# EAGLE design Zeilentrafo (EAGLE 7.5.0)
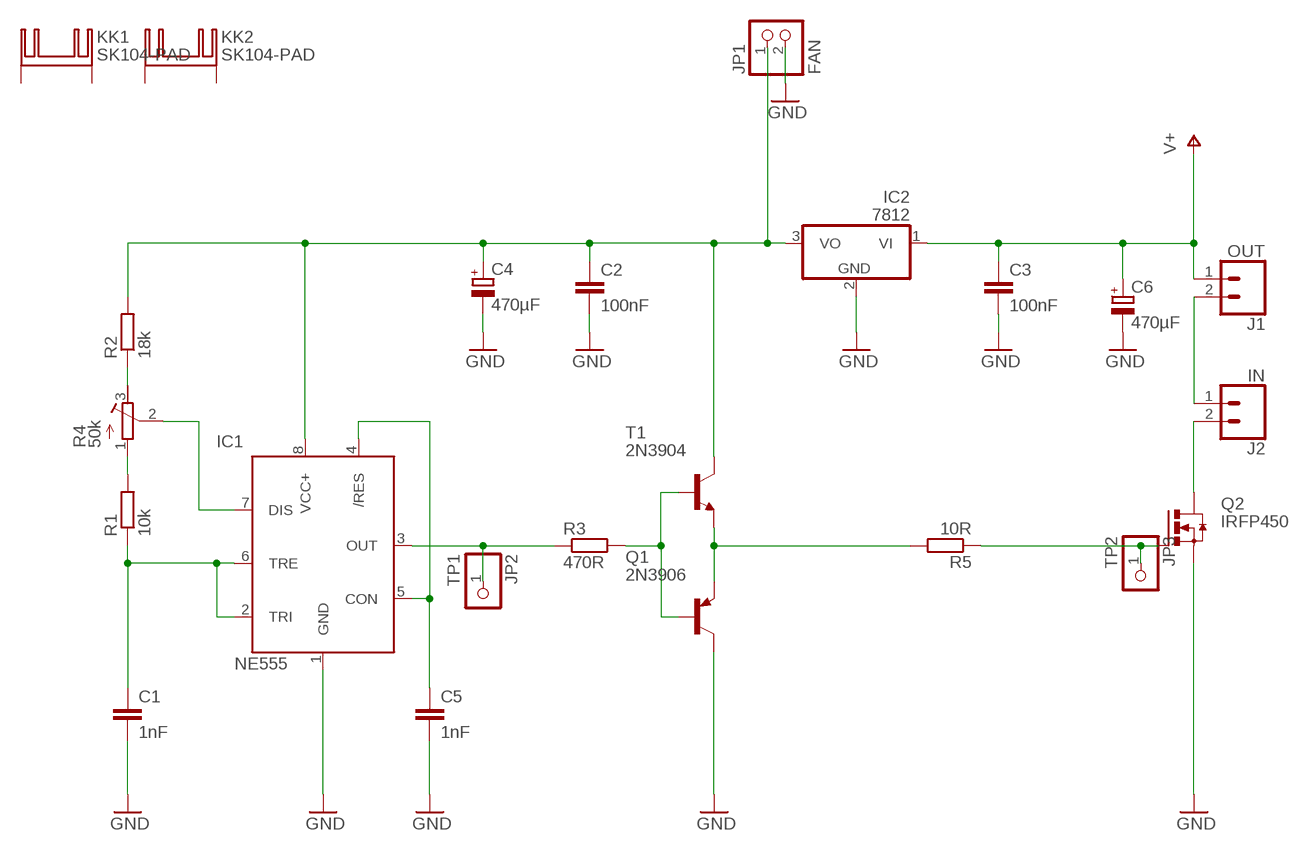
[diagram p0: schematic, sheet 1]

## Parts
C1  1nF  C-EU050-024X044  [C050-024X044]
C2  100nF  C-EU050-024X044  [C050-024X044]
C3  100nF  C-EU050-024X044  [C050-024X044]
C4  470µF  CPOL-EUE5-10.5  [E5-10,5]
C5  1nF  C-EU050-024X044  [C050-024X044]
C6  470µF  CPOL-EUE5-10.5  [E5-10,5]
IC1  NE555  [DIL-08]
IC2  7812  7812TV  [TO220V]
J1  OUT  CONN_025MM  [SCREWTERMINAL-5MM-2]
J2  IN  CONN_025MM  [SCREWTERMINAL-5MM-2]
JP1  FAN  PINHD-1X2  [1X02]
JP2  TP1  PINHD-1X1  [1X01]
JP3  TP2  PINHD-1X1  [1X01]
KK1  SK104-PAD  [SK104-PAD]
KK2  SK104-PAD  [SK104-PAD]
Q1  2N3906  [TO92]
Q2  IRFP450  IRFP240  [TO247BV]
R1  10k  R-EU_0207/12  [0207/12]
R2  18k  R-EU_0207/12  [0207/12]
R3  470R  R-EU_0207/12  [0207/12]
R4  50k  R-TRIMM3296Y  [RTRIM3296Y]
R5  10R  R-EU_0207/12  [0207/12]
T1  2N3904  [TO92]

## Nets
GND: C1.2 C2.2 C3.2 C4.- C5.2 C6.- IC1.1(GND) IC2.2(GND) JP1.2 Q1.1(C) Q2.S
N$1: C1.1 IC1.2(TRI) IC1.6(TRE) R1.1
N$2: IC1.7(DIS) R4.2(S)
N$3: R1.2 R4.1(A)
N$4: R2.1 R4.3(E)
N$5: C2.1 C4.+ IC1.8(VCC+) IC2.3(VO) JP1.1 R2.2 T1.1(C)
N$6: JP3.1 Q2.G R5.1
N$7: IC1.3(OUT) JP2.1 R3.1
N$8: Q1.2(B) R3.2 T1.2(B)
N$9: Q1.3(E) R5.2 T1.3(E)
N$10: J1.2 J2.1
N$11: C5.1 IC1.4(/RES) IC1.5(CON)
N$13: J2.2 Q2.D
V+: C3.1 C6.+ IC2.1(VI) J1.1
Unconnected: KK1.K1(K) KK1.K2(K) KK2.K1(K) KK2.K2(K)

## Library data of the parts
C1-C3 C5 = rcl_custom:C-EU: CAPACITOR, European symbol
C4 C6 = rcl_custom:CPOL-EU: POLARIZED CAPACITOR, European symbol
IC1 = st-microelectronics_custom:NE555: General purpose bipolar Timer; MF: Arrow Electronics; MPN: NE555N; OC_FARNELL: 1467742; OC_NEWARK: 89K1486
IC2 = linear:78*: Positive VOLTAGE REGULATOR Source: http://cache.national.com/ds/LM/LM78L05.pdf http://www.fairchildsemi.com/ds/LM/LM7805.pdf
J1 J2 = SparkFun-Connectors:CONN_02: Multi connection point. Often used as Generic Header-pin footprint for 0.1 inch spaced/style header connections; SF_SKU: PRT-08432
JP1 = pinhead:PINHD-1X2: PIN HEADER
JP2 JP3 = pinhead:PINHD-1X1: PIN HEADER
KK1 KK2 = heatsink_custom:SK104-PAD: HEATSINK
Q1 = transistor-pnp:2N3906: PNP Transistor
Q2 = transistor-power:IRFP240: HEXFET Power MosFet Source: http://www.irf.com/
R1-R3 R5 = rcl_custom:R-EU_: RESISTOR, European symbol
R4 = rcl:R-TRIMM: Trimm resistor
T1 = transistor:2N3904: NPN TRANSISTOR

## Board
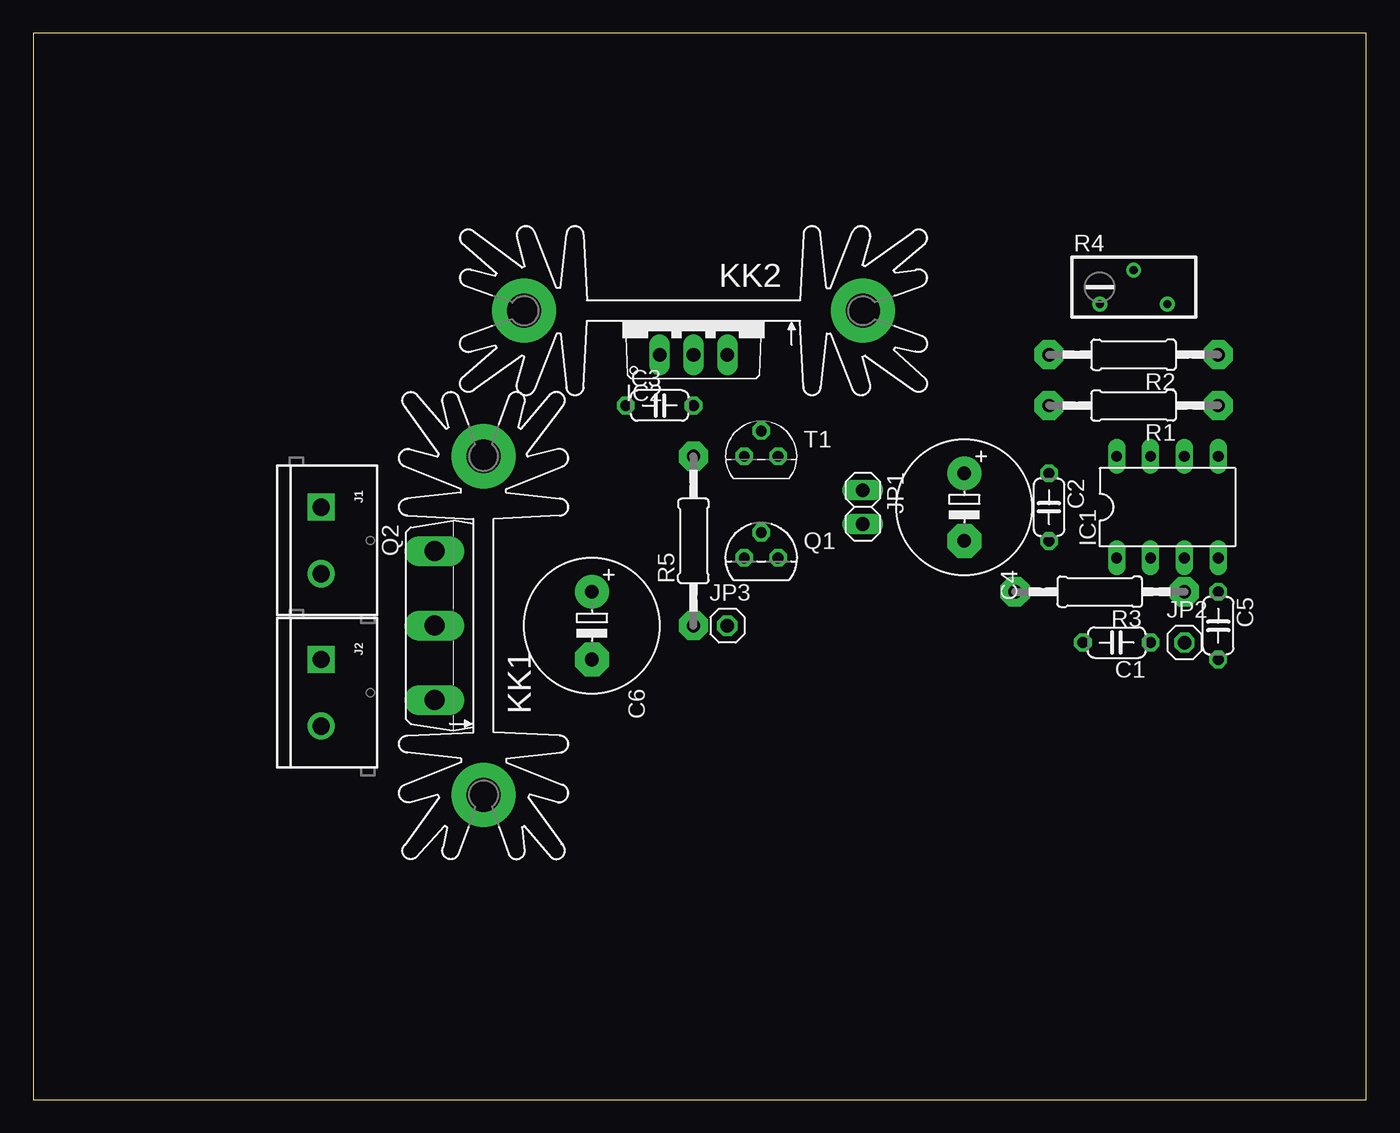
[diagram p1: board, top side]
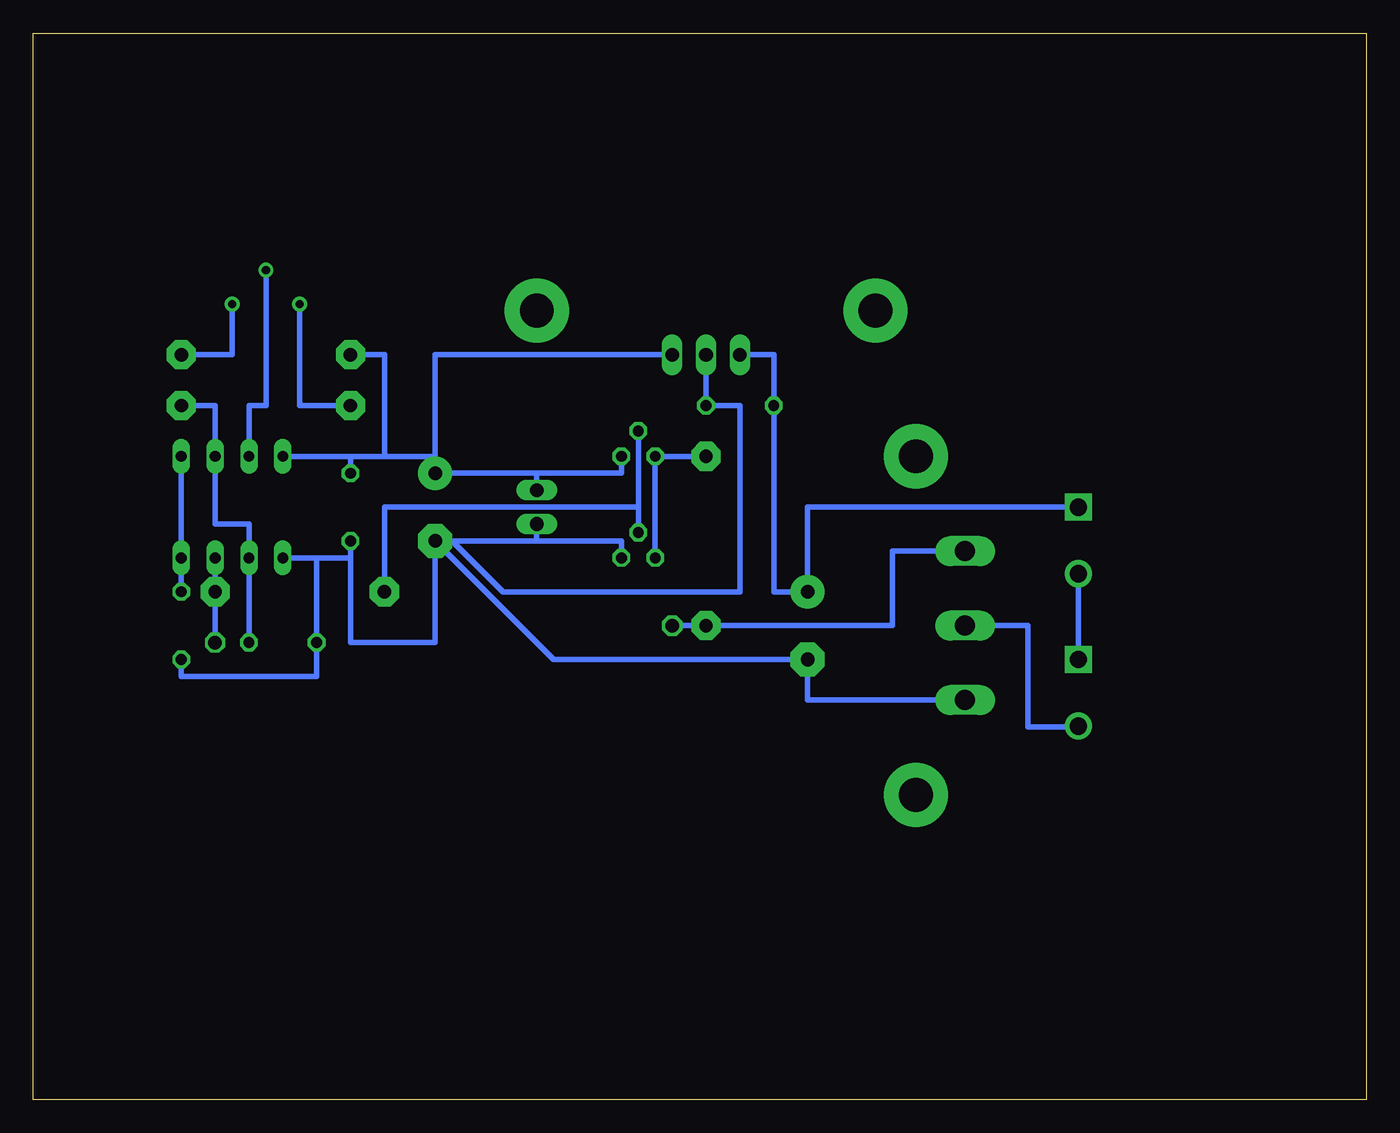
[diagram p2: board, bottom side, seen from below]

Size 100 x 80 mm. Coordinates in mm from the lower left corner, seen from the top.
Outline: 0,0 100,0 100,80 0,80 0,0
Copper layers (1*16): Top 0.035mm / dielectric 1.5mm / Bottom 0.035mm
Design rules "default": minimum track width 10mil, minimum drill 24mil, track to track 8mil, track to pad 8mil, pad to pad 8mil, via to via 8mil, smd to smd 8mil, copper to edge 40mil, drill to drill 8mil, minimum pad ring 10mil, minimum via ring 8mil, stop-mask expansion 4mil, vias tented up to drill 0mil, thermal gap 10mil

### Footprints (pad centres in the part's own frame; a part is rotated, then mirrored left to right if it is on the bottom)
C050-024X044 = drill 0.813 octagon: 1 -2.54,0; 2 2.54,0
E5-10,5 = drill 1.016 pad 2.54: + -2.54,0 | drill 1.016 pad 2.54 octagon: - 2.54,0
DIL-08 = drill 0.813 long: 1 -3.81,-3.81; 2 -1.27,-3.81; 3 1.27,-3.81; 4 3.81,-3.81; 5 3.81,3.81; 6 1.27,3.81; 7 -1.27,3.81; 8 -3.81,3.81
TO220V = drill 1.016 long: 1 -2.54,-2.54; 2 0,-2.54; 3 2.54,-2.54
SCREWTERMINAL-5MM-2 = drill 1.3 pad 2.032 square: 1 0,0 | drill 1.3 pad 2.032: 2 5,0
1X02 = drill 1.016 long: 1 -1.27,0; 2 1.27,0
1X01 = drill 1.016 octagon: 1 0,0
SK104-PAD = drill 2.54 pad 4.81: K1 -12.7,-0.762; K2 12.7,-0.762
TO92 = drill 0.813 octagon: 1 1.27,0; 2 0,1.905; 3 -1.27,0
TO247BV = drill 1.499 long: D 0,-2.921; G -5.588,-2.921; S 5.588,-2.921
0207/12 = drill 1 pad 2.184 octagon: 1 -6.35,0; 2 6.35,0
RTRIM3296Y = drill 0.61: 1 1.27,-2.54; 2 -1.27,0; 3 1.27,2.54

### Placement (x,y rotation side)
C1  81.28,34.29 180 top
C2  76.2,44.45 270 top
C3  46.99,52.07 0 top
C4  69.85,44.45 270 top
C5  88.9,35.56 270 top
C6  41.91,35.56 270 top
IC1  85.09,44.45 0 top
IC2  49.53,58.42 0 top
J1  21.59,44.45 270 top
J2  21.59,33.02 270 top
JP1  62.23,44.45 270 top
JP2  86.36,34.29 0 top
JP3  52.07,35.56 0 top
KK1  33.02,35.56 90 top
KK2  49.53,58.42 180 top
Q1  54.61,40.64 0 top
Q2  33.02,35.56 270 top
R1  82.55,52.07 180 top
R2  82.55,55.88 180 top
R3  80.01,38.1 180 top
R4  82.55,60.96 270 top
R5  49.53,41.91 90 top
T1  54.61,48.26 0 top

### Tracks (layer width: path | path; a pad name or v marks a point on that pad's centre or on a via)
GND
  Bottom 0.406: IC1.1 78.74,40.64 | 78.74,40.64 76.2,40.64 | 78.74,40.64 C1.2 78.74,31.75 88.9,31.75 C5.2 | C2.2 76.2,40.64 | JP1.2 62.23,41.91 | 62.23,41.91 68.58,41.91 | 68.58,41.91 C4.- | Q1.1 55.88,41.91 62.23,41.91 | C4.- 69.85,34.29 76.2,34.29 76.2,40.64 | IC2.2 C3.2 46.99,52.07 46.99,38.1 64.77,38.1 68.58,41.91 | Q2.S 41.91,29.97 C6.- 60.96,33.02 C4.-
N$1
  Bottom 0.406: C1.1 IC1.2 83.82,43.18 86.36,43.18 IC1.6 86.36,52.07 R1.1
N$2
  Bottom 0.406: IC1.7 83.82,52.07 82.55,52.07 R4.2
N$3
  Bottom 0.406: R1.2 80.01,52.07 R4.1
N$4
  Bottom 0.406: R4.3 85.09,55.88 R2.1
N$5
  Bottom 0.406: IC1.8 76.2,48.26 | 76.2,48.26 73.66,48.26 | 73.66,48.26 69.85,48.26 C4.+ | C2.1 76.2,48.26 | JP1.1 62.23,46.99 | 62.23,46.99 C4.+ | R2.2 73.66,55.88 73.66,48.26 | IC2.3 69.85,55.88 C4.+ | T1.1 55.88,46.99 62.23,46.99
N$6
  Bottom 0.406: JP3.1 R5.1 35.56,35.56 35.56,41.15 Q2.G
N$7
  Bottom 0.406: IC1.3 R3.1 JP2.1
N$8
  Bottom 0.406: T1.2 54.61,44.45 | 54.61,44.45 Q1.2 | R3.2 73.66,44.45 54.61,44.45
N$9
  Bottom 0.406: Q1.3 T1.3 R5.2
N$10
  Bottom 0.406: J1.2 J2.1
N$11
  Bottom 0.406: IC1.5 IC1.4 C5.1
N$13
  Bottom 0.406: J2.2 21.59,27.94 25.4,27.94 25.4,35.56 Q2.D
V+
  Bottom 0.406: IC2.1 44.45,55.88 C3.1 44.45,38.1 C6.+ 41.91,44.45 J1.1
